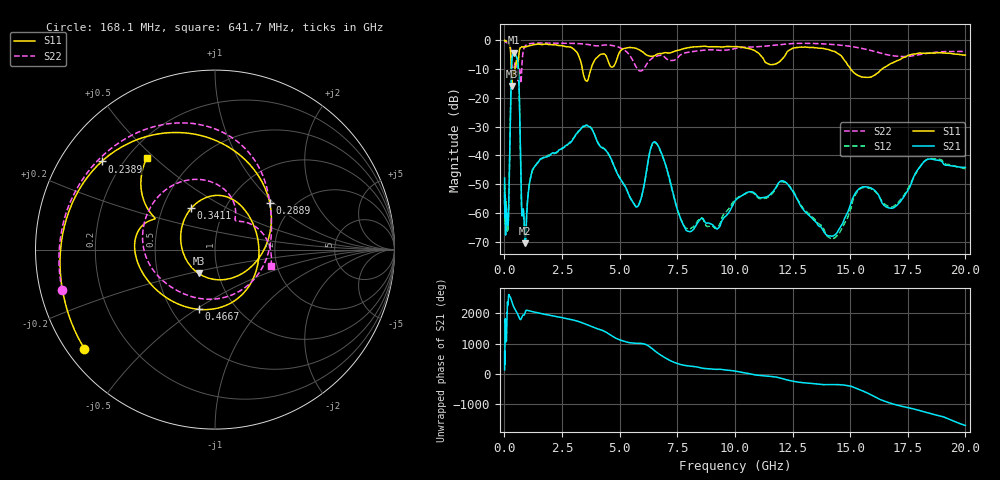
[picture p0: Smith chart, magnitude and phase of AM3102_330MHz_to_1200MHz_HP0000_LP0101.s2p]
! Date/Time: Tue, Sep 11, 2018 5:08 PM
! Network Analyzer: Agilent Technologies E8362B Rev: A.07.50.63
! Sweep from 0.010 to 20.000 GHz, 1601 Points, Sweep Type: LOG
! Power Supply: 4.950 V, 0.001 A
# Hz S DB R 50
!freq MagS11 AngS11 MagS21 AngS21 MagS12 AngS12 MagS22 AngS22
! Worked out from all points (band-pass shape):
!   1601 points, 10 MHz to 20 GHz, reference 50 ohm
!   highest |S21| = -4.26 dB at 412.5 MHz (marker M1); lowest = -70.5 dB at 907.7 MHz (marker M2)
!   |S21| within 3 dB of the highest: 320.6 MHz to 584.4 MHz (263.8 MHz wide, 58.3 % of centre)
!   lowest |S11| = -15.9 dB at 316.2 MHz (marker M3), VSWR 1.38, Z = 40.3 - j11 ohm
!   |S11| at or under -10 dB: 294.7 MHz to 450.4 MHz (155.7 MHz wide, 41.8 % of centre); 3.383 GHz to 3.757 GHz (374.2 MHz wide, 10.5 % of centre); 15.03 GHz to 16.38 GHz (1.352 GHz wide, 8.61 % of centre)
!   |S22| runs from -14.8 to -0.2 dB; largest |S21 - S12| = 0.01
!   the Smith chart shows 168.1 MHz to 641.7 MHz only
!   S11 on the Smith chart (normalised r, x): 168.1 MHz: 0.05, -0.34; 238.9 MHz: 0.12, +0.34; 288.9 MHz: 1.52, +0.95; 341.1 MHz: 0.70, +0.34; 466.7 MHz: 0.68, -0.51; 641.7 MHz: 0.27, +0.47
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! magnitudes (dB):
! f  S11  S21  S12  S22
! 10 MHz  0.0  -47.9  -57.4  -0.2
! 35.55 MHz  0.0  -59.9  -58.9  -0.4
! 126.4 MHz  -0.4  -63.3  -64.6  -0.9
! 168.1 MHz  -0.8  -62.7  -63.4  -1.1
! 238.9 MHz  -1.9  -36.1  -36.2  -1.8
! 288.9 MHz  -7.9  -14.7  -14.7  -4.0
! 316.2 MHz  -15.9  -7.8  -7.9  -7.5
! 341.1 MHz  -11.5  -5.7  -5.8  -10.2
! 412.5 MHz  -12.2  -4.3  -4.3  -9.8
! 447.2 MHz  -10.2  -4.5  -4.5  -8.2
! 466.7 MHz  -9.2  -4.7  -4.7  -7.7
! 641.7 MHz  -3.9  -17.4  -17.5  -9.8
! 750.6 MHz  -2.2  -59.1  -58.9  -10.4
! 907.7 MHz  -2.3  -70.5  -71.5  -1.9
! 1.59 GHz  -1.4  -41.1  -41.2  -0.9
! 3.634 GHz  -13.6  -29.7  -29.5  -1.4
! 5.652 GHz  -2.6  -57.2  -57.3  -8.2
! 6.58 GHz  -5.0  -35.6  -35.7  -5.5
! 7.958 GHz  -2.5  -66.3  -65.5  -4.1
! 12.09 GHz  -6.1  -48.9  -49.2  -1.3
! 14.21 GHz  -3.6  -68.1  -69.0  -1.4
! 20 GHz  -5.1  -44.2  -44.6  -3.8
